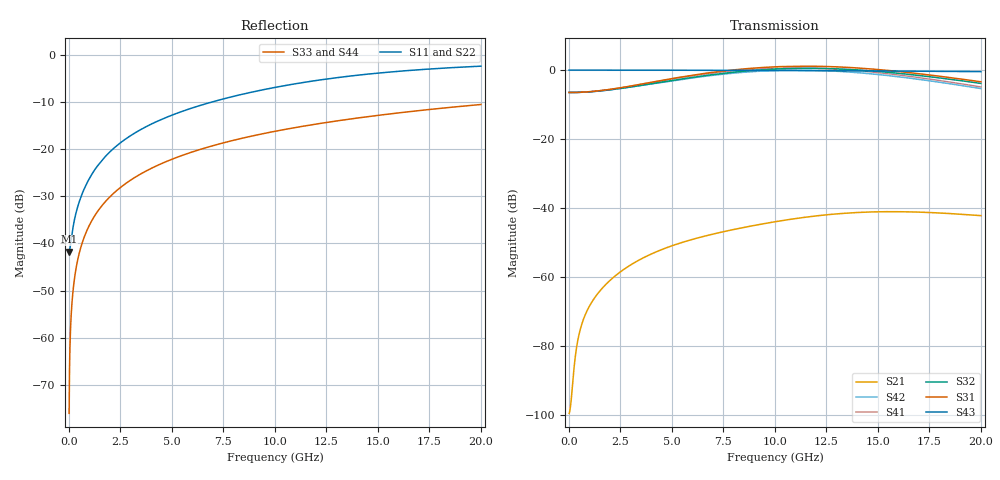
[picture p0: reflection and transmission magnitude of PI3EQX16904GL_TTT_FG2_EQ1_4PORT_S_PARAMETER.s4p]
! NPort=4 DATA=2000 NOISE=0 GROUPDELAY=0 COMPLEX_DATAFORMAT=POLAR
! NumOfBlock=1 NumOfParam=0
! .MODEL Smodel S TSTONEFILE=PI3EQX16904GL_TTT_FG2_EQ1_4PORT_S_PARAMETER.s4p TYPE=S
!  -- The above .MODEL line can be used for the S element in the netlist.
! The s parameter is extracted from the linear redriver, it is not bi-directional; only s(4,1)s(4,2) and s(3,1)s(3,2)
! should be the insertion loss
!Port definition:
!Port1 = input+
!Port2 = input-
!Port3 = output+
!Port4 = output-
# Hz S MA R  50
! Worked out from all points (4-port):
!   2000 points, 10 MHz to 20 GHz, reference 50 ohm
!   strongest paths, dB at 10 MHz, 5.01 GHz, 10.01 GHz, 15.01 GHz, 20 GHz:
!     S43: 0.0, 0.0, -0.1, -0.3, -0.4
!     S31: -6.5, -2.4, 1.0, 0.2, -3.4
!     S32: -6.5, -3.0, 0.3, -0.4, -3.9
!     S41: -6.5, -2.6, 0.5, -0.7, -4.9
!     S42: -6.5, -3.1, -0.1, -1.3, -5.4
!     S21: -99.6, -51.0, -44.0, -41.1, -42.2
!   lowest |S11| = -41.7 dB at 10 MHz (marker M1), VSWR 1.02, Z = 49.2 - j0.0603 ohm
!   |S11| at or under -10 dB: start of sweep to 6.916 GHz
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1e7  0.008182 -175.7  1.049e-05 7.4  0 0.0  0 0.0
     1.049e-05 7.4  0.008182 -175.7  0 0.0  0 0.0
     0.4742 -0.1  0.4742 179.9  0.0001571 -90.0  1 -0.0
     0.4742 179.9  0.4742 -0.1  1 -0.0  0.0001571 -90.0
2e8  0.01483 -130.6  3.32e-05 105.3  0 0.0  0 0.0
     3.32e-05 105.3  0.01483 -130.6  0 0.0  0 0.0
     0.4741 -0.3  0.474 179.5  0.003142 -90.2  1 -0.2
     0.4741 179.4  0.474 -0.9  1 -0.2  0.003142 -90.2
6.2e8  0.03268 -112.4  0.0002037 112.9  0 0.0  0 0.0
       0.0002037 112.9  0.03268 -112.4  0 0.0  0 0.0
       0.478 -0.6  0.4771 178.7  0.009738 -90.6  0.9999 -0.6
       0.4779 178.3  0.477 -2.4  0.9999 -0.6  0.009738 -90.6
2.97e9  0.1383 -101.7  0.001474 93.6  0 0.0  0 0.0
        0.001475 93.5  0.1383 -101.7  0 0.0  0 0.0
        0.5854 -8.1  0.5683 169.5  0.0466 -92.8  0.9988 -2.7
        0.5828 166.6  0.5658 -15.8  0.9988 -2.7  0.0466 -92.8
1.055e10  0.4768 -114.3  0.006757 38.0  0 0.0  0 0.0
          0.006701 38.0  0.4757 -114.4  0 0.0  0 0.0
          1.131 -101.1  1.052 79.2  0.1633 -99.8  0.9855 -9.4
          1.071 60.6  0.9965 -119.1  0.9855 -9.4  0.1633 -99.8
1.465e10  0.6319 -124.2  0.008792 1.9  0 0.0  0 0.0
          0.008747 2.3  0.63 -124.2  0 0.0  0 0.0
          1.04 -164.8  0.9769 16.0  0.2238 -103.5  0.9726 -12.9
          0.9418 -9.5  0.8843 171.3  0.9726 -12.9  0.2238 -103.5
2e10  0.7622 -135.5  0.007778 -37.3  0 0.0  0 0.0
      0.007737 -37.1  0.7608 -135.4  0 0.0  0 0.0
      0.6773 122.2  0.6415 -56.8  0.2986 -108.1  0.9506 -17.4
      0.5703 -89.7  0.5401 91.3  0.9506 -17.4  0.2986 -108.1
